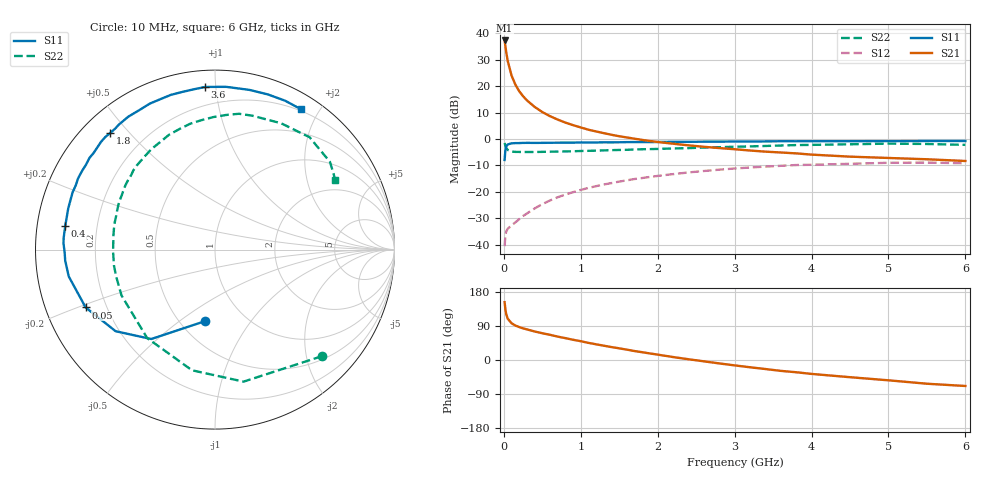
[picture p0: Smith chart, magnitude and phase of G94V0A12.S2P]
! SIEMENS Small Signal Semiconductors
! BFG235
! Si NPN RF Bipolar Junction Transistor in SOT223
! VCE = 4 V  IC = 120 mA
! Common Emitter S-Parameters:  July  1994
# GHz  S  MA  R  50
!  f  S11  S21  S12  S22
! GHz  MAG  ANG  MAG  ANG  MAG  ANG  MAG  ANG
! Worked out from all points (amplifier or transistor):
!   40 points, 10 MHz to 6 GHz, reference 50 ohm
!   highest |S21| = 37.3 dB at 10 MHz (marker M1)
!   |S21| within 3 dB of that: start of sweep to 24.34 MHz
!   unconditionally stable (mu >= 1): 462.4 MHz to 1.509 GHz
!   at 200 MHz: K = 0.80, MSG = 24.2 dB, |S12| = -30.3 dB
!   at 1.5 GHz: K = 1.00, MAG = 8.3 dB, |S12| = -16.1 dB
!   at 6 GHz: K = 0.90, MSG = 0.4 dB, |S12| = -9.2 dB
!   S11 on the Smith chart (normalised r, x): 10 MHz: 0.66, -0.63; 50 MHz: 0.12, -0.21; 400 MHz: 0.08, +0.08; 1.8 GHz: 0.08, +0.44; 3.6 GHz: 0.09, +0.94; 6 GHz: 0.18, +1.77
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0.01  0.4014 -97.6  73.15 152.6  0.0094 63.1  0.8412 -44.9
0.02  0.612 -125.5  57.49 133.7  0.0146 49.1  0.7527 -77.8
0.03  0.7164 -140.6  45.2 121.8  0.0177 41.7  0.6844 -100.8
0.05  0.7896 -155.9  30.14 109.2  0.02 33.5  0.621 -127.5
0.1  0.8284 -169.6  15.91 97.0  0.0233 35.5  0.5802 -153.9
0.15  0.8369 -175.8  10.7 90.9  0.0265 42.2  0.5706 -164.8
0.2  0.838 -179.2  8.01 86.9  0.0305 46.6  0.5699 -171.0
0.25  0.8444 177.9  6.452 83.5  0.035 50.1  0.5675 -175.2
0.3  0.8457 175.7  5.392 80.8  0.039 53.3  0.568 -178.8
0.4  0.8447 171.1  4.054 75.3  0.0486 55.9  0.5681 176.1
0.5  0.8455 167.6  3.238 70.6  0.0587 57.3  0.5714 171.9
0.7  0.8515 160.8  2.332 61.7  0.0792 57.1  0.5791 164.5
0.9  0.8544 155.2  1.829 53.4  0.0988 54.4  0.5869 158.3
1.1  0.8609 149.1  1.5 45.2  0.1187 51.2  0.5981 152.2
1.4  0.8643 141.7  1.202 34.1  0.1469 45.3  0.6156 143.8
1.8  0.8734 132.0  0.961 20.5  0.183 36.8  0.6401 132.9
2.2  0.8842 123.1  0.815 7.8  0.2168 27.9  0.663 122.2
3.2  0.8971 101.7  0.606 -19.2  0.2891 4.6  0.7249 96.1
3.6  0.9077 93.5  0.556 -28.7  0.3112 -5.2  0.7532 85.1
4.5  0.9103 77.8  0.464 -45.4  0.3399 -25.0  0.7946 62.3
5.5  0.9169 64.8  0.414 -62.6  0.358 -46.9  0.8055 37.3
6  0.917 58.6  0.384 -68.6  0.3481 -55.1  0.775 30.1
